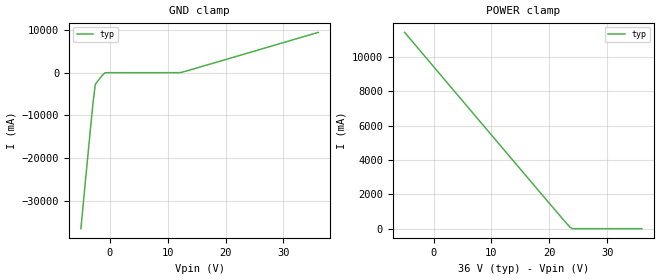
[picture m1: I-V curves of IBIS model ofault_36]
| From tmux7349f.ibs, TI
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| ofault_36
[Model]   ofault_36
Model_type   Input
Vinl = 0.8
Vinh = 1.3
|   typ   min   max
C_comp   2.533030e-12   NA   NA
[Voltage Range]   36   NA   NA
[Temperature Range]   27   NA   NA
[Power Clamp Reference]   36   NA   NA
[GND Clamp Reference]   0   NA   NA
[GND Clamp]
|   Voltage   I(typ)   I(min)   I(max)
-5V       -36.55A    NA         NA
-3.758V   -18.93A    NA         NA
-2.929V   -7.435A    NA         NA
-2.515V   -2.769A    NA         NA
-858.6mV  -42.96mA   NA         NA
12.39V    73.42mA    NA         NA
36V       9.435A     NA         NA
[POWER Clamp]
|   Voltage   I(typ)   I(min)   I(max)
-5V       11.43A     NA         NA
23.58V    84.1mA     NA         NA
23.99V    35.46uA    NA         NA
36V       0A         NA         NA
